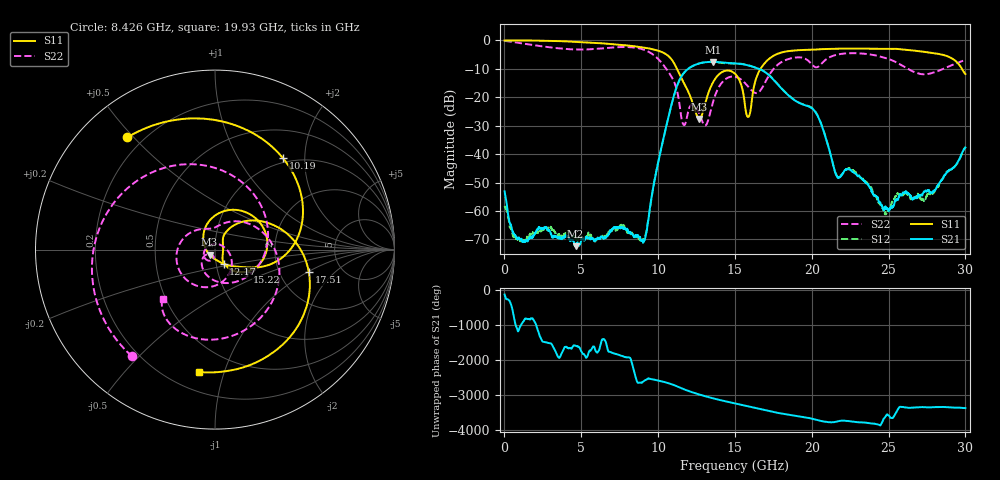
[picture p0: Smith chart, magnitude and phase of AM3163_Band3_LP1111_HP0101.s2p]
!Agilent Technologies,E8364B,MY43040894,A.07.50.67
!Agilent E8364B: A.07.50.67
!Date: Thursday, August 20, 2020 12:16:21
!Correction: S11(Full 2 Port(1,2))
!S21(Full 2 Port(1,2))
!S12(Full 2 Port(1,2))
!S22(Full 2 Port(1,2))
!S2P File: Measurements: S11, S21, S12, S22:
# Hz S  dB  R 50
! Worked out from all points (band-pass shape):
!   3201 points, 10 MHz to 30 GHz, reference 50 ohm
!   highest |S21| = -7.52 dB at 13.56 GHz (marker M1); lowest = -72.3 dB at 4.63 GHz (marker M2)
!   |S21| within 3 dB of the highest: 11.84 GHz to 16.78 GHz (4.945 GHz wide, 34.6 % of centre)
!   lowest |S11| = -27.6 dB at 12.68 GHz (marker M3), VSWR 1.09, Z = 47 - j2.69 ohm
!   |S11| at or under -10 dB: 11.23 GHz to 16.66 GHz (5.436 GHz wide, 39 % of centre); 29.78 GHz to end of sweep
!   |S22| runs from -29.9 to -0.2 dB; largest |S21 - S12| = 0.012
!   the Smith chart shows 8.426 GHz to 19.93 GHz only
!   S11 on the Smith chart (normalised r, x): 8.426 GHz: 0.14, +0.48; 10.19 GHz: 0.93, +1.58; 12.17 GHz: 1.09, -0.17; 15.22 GHz: 1.39, -0.36; 17.51 GHz: 2.92, -1.02; 19.93 GHz: 0.32, -0.83
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1e7  -0.02 -2.1  -53.07 -142.7  -58.16 123.8  -0.15 -5.2
1.218972e9  -0.01 -33.2  -70.92 175.0  -70.48 -4.0  -1.10 -80.8
2.55915e9  -0.09 -69.6  -66.13 -47.1  -66.44 -149.4  -2.15 -157.7
4.630334e9  -0.48 -124.2  -72.35 -157.3  -69.80 -175.0  -3.17 93.1
5.014581e9  -0.58 -134.3  -69.88 32.2  -69.78 162.3  -3.20 72.5
6.635916e9  -1.12 -177.7  -69.01 -112.1  -68.37 64.8  -2.68 -18.5
8.425944e9  -2.01 128.1  -69.07 -142.2  -68.15 -133.2  -2.46 -128.0
9.138206e9  -2.54 102.1  -70.00 -61.6  -69.03 56.8  -3.39 -179.9
1.000979e10  -3.61 62.9  -42.74 -65.4  -42.61 -64.8  -6.54 96.4
1.018786e10  -3.95 53.3  -38.31 -83.0  -38.28 -82.9  -7.59 73.9
1.216532e10  -20.70 -58.8  -9.23 -28.8  -9.24 -28.4  -22.70 -126.7
1.268078e10  -27.57 -136.8  -8.08 -100.8  -8.06 -100.5  -25.73 174.8
1.356173e10  -14.86 93.6  -7.52 152.3  -7.59 151.8  -21.80 -13.2
1.5005e10  -11.70 -18.6  -8.07 5.5  -8.14 7.2  -12.77 -149.7
1.522055e10  -13.23 -34.1  -8.16 -15.4  -8.15 -13.7  -13.16 -168.1
1.587658e10  -26.87 3.8  -8.79 -79.3  -8.72 -78.6  -16.31 135.7
1.750729e10  -5.40 -13.4  -13.80 121.3  -13.69 122.0  -10.06 7.7
1.992523e10  -3.25 -97.4  -23.55 -58.7  -23.38 -57.9  -7.95 -136.6
2.000958e10  -3.24 -99.5  -23.84 -67.5  -23.68 -66.9  -8.44 -137.8
2.500479e10  -2.99 144.5  -60.09 25.6  -59.72 155.1  -6.55 67.8
2.740399e10  -4.07 76.9  -52.76 -102.8  -55.84 -94.6  -11.89 -88.4
3e10  -11.82 -29.4  -37.66 -129.5  -37.48 -130.6  -6.93 130.4
